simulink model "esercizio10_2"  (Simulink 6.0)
settings: Solver=ode45  StartTime=0.0  StopTime=4*pi  RelTol=1e-3

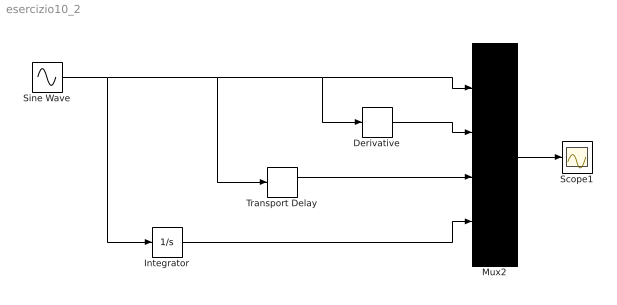
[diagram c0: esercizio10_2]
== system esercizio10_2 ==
  Derivative : Derivative
  Integrator : Integrator
  Mux2 : Mux
  Scope1 : Scope
  Sine Wave : Sin  Frequency=2  SampleTime=0
  Transport Delay : TransportDelay  DelayTime=pi/2
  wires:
  Mux2/1 -> Scope1/1
  Sine Wave/1 -> Mux2/1, Derivative/1, Transport Delay/1, Integrator/1
  Derivative/1 -> Mux2/2
  Integrator/1 -> Mux2/4
  Transport Delay/1 -> Mux2/3
